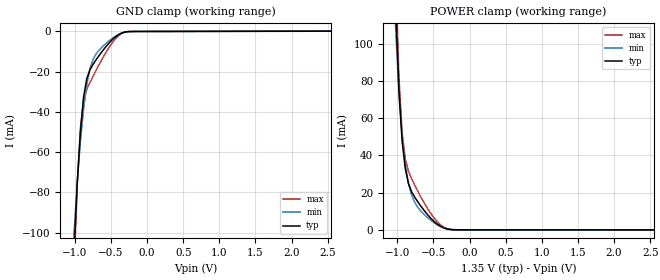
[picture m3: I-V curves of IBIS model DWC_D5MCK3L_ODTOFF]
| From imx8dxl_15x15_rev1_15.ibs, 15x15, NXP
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[Model] DWC_D5MCK3L_ODTOFF
Model_type   Input
Polarity   Non-Inverting
Enable   Active-High
C_comp   1.262pF   1.180pF   1.365pF
C_comp_power_clamp   279.441fF   258.852fF   306.885fF
C_comp_gnd_clamp 973.651fF   908.565fF   1.053pF
Vinh = 800.000mV
Vinl = 550.000mV
[Model Spec]
D_overshoot_ampl_h 0.4 NA   NA
D_overshoot_ampl_l 0.4 NA   NA
D_overshoot_area_l 100.000p NA   NA
D_overshoot_area_h 100.000p NA   NA
[Receiver Thresholds]
Vcross_low = 525.000mV
Vcross_high = 825.000mV
Vdiff_ac = 250.000mV
Vdiff_dc = 180.000mV
Tdiffslew_ac = 10.000ns
[Temperature Range]   25.000   125.000   -40.000
[Voltage Range]   1.350V   1.283V   1.450V
[GND Clamp Reference]   0.00V   0.00V   0.00V
[C Comp Corner]
| variable   typ   min   max
C_comp 1.262pF   1.365pF   1.180pF
C_comp_pullup 279.441fF   306.885fF   258.852fF
C_comp_pulldown 973.651fF   1.053pF   908.565fF
[POWER Clamp Reference]   1.350V   1.283V   1.450V
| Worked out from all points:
|   GND clamp passes 1 mA (typ) near -0.36 V on its own axis
|   POWER clamp passes 1 mA (typ) near -0.36 V on its own axis
[GND Clamp]
-1.318V   -593.4mA   -427mA     -758.7mA
-1.011V   -108.7mA   -99.8mA    -118.2mA
-966.7mV  -74.7mA    -74.6mA    -75.87mA
-922.7mV  -49.41mA   -54.3mA    -47.9mA
-878.8mV  -32.42mA   -38.21mA   -34.12mA
-834.8mV  -23.33mA   -26.23mA   -28.72mA
-790.9mV  -19.01mA   -18.35mA   -25.26mA
-747mV    -16.25mA   -13.76mA   -22.11mA
-483.3mV  -4.093mA   -3.434mA   -5.633mA
-351.5mV  -766.8uA   -911.3uA   -894.7uA
-263.6mV  -79.41uA   -192.1uA   -51.43uA
2.68V     154.9uA    127.3uA    193.1uA
[Power Clamp]
-1.33V    727.8mA    510.6mA    954.1mA
-1.023V   119.4mA    107.4mA    137.5mA
-978.8mV  74.87mA    74.2mA     82.23mA
-934.8mV  47.95mA    50.66mA    52.21mA
-890.9mV  32.9mA     35.12mA    38.1mA
-847mV    24.9mA     25.11mA    31.53mA
-759.1mV  17.5mA     14.71mA    23.9mA
-671.2mV  12.54mA    9.915mA    17.38mA
-495.5mV  4.603mA    3.922mA    6.563mA
-363.6mV  1.088mA    1.21mA     1.541mA
-231.8mV  46.56uA    141.4uA    53.69uA
2.668V    -76.24uA   -66.58uA   -87.76uA
